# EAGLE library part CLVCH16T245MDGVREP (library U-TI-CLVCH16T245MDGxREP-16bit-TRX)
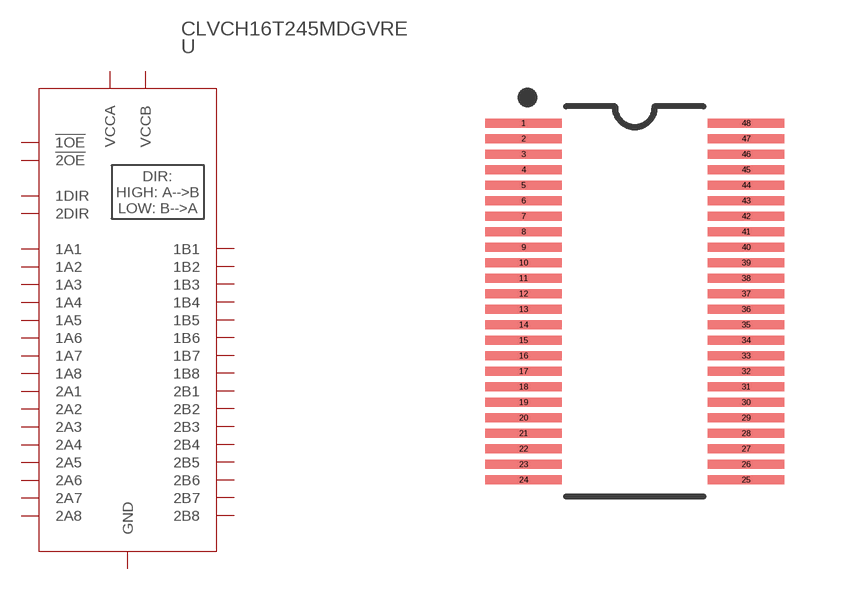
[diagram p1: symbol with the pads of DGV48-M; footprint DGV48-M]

Designator prefix U

## CLVCH16T245MDGVREPDGV48-M (MANUFACTURER_PART_NUMBER: CLVCH16T245MDGVREP; VENDOR: Texas Instruments)  [DGV48-M]
1  1DIR  in
2  1B1
3  1B2
4  GND  pwr
5  1B3
6  1B4
7  VCCB  pwr
8  1B5
9  1B6
10  GND  pwr
11  1B7
12  1B8
13  2B1
14  2B2
15  GND  pwr
16  2B3
17  2B4
18  VCCB  pwr
19  2B5
20  2B6
21  GND  pwr
22  2B7
23  2B8
24  2DIR  in
25  !2OE  in
26  2A8
27  2A7
28  GND  pwr
29  2A6
30  2A5
31  VCCA  pwr
32  2A4
33  2A3
34  GND  pwr
35  2A2
36  2A1
37  1A8
38  1A7
39  GND  pwr
40  1A6
41  1A5
42  VCCA  pwr
43  1A4
44  1A3
45  GND  pwr
46  1A2
47  1A1
48  !1OE  in

## Footprint DGV48-M (pad centres in mm)
smd 1.981 x 0.229: 1 -2.87,4.6; 2 -2.87,4.2; 3 -2.87,3.8; 4 -2.87,3.4; 5 -2.87,3; 6 -2.87,2.6; 7 -2.87,2.2; 8 -2.87,1.8; 9 -2.87,1.4; 10 -2.87,1; 11 -2.87,0.6; 12 -2.87,0.2; 13 -2.87,-0.2; 14 -2.87,-0.6; 15 -2.87,-1; 16 -2.87,-1.4; 17 -2.87,-1.8; 18 -2.87,-2.2; 19 -2.87,-2.6; 20 -2.87,-3; 21 -2.87,-3.4; 22 -2.87,-3.8; 23 -2.87,-4.2; 24 -2.87,-4.6; 25 2.87,-4.6; 26 2.87,-4.2; 27 2.87,-3.8; 28 2.87,-3.4; 29 2.87,-3; 30 2.87,-2.6; 31 2.87,-2.2; 32 2.87,-1.8; 33 2.87,-1.4; 34 2.87,-1; 35 2.87,-0.6; 36 2.87,-0.2; 37 2.87,0.2; 38 2.87,0.6; 39 2.87,1; 40 2.87,1.4; 41 2.87,1.8; 42 2.87,2.2; 43 2.87,2.6; 44 2.87,3; 45 2.87,3.4; 46 2.87,3.8; 47 2.87,4.2; 48 2.87,4.6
